{attribute 'TcGenerated'}
{attribute 'no-analysis'}
// This function has been automatically generated from the project information.
VAR_GLOBAL CONSTANT
	{attribute 'const_non_replaced'}
	{attribute 'linkalways'}
	stLibVersion_test : ST_LibVersion := (iMajor := 0, iMinor := 0, iBuild := 0, iRevision := 0, sVersion := '0.0.0');
END_VAR
